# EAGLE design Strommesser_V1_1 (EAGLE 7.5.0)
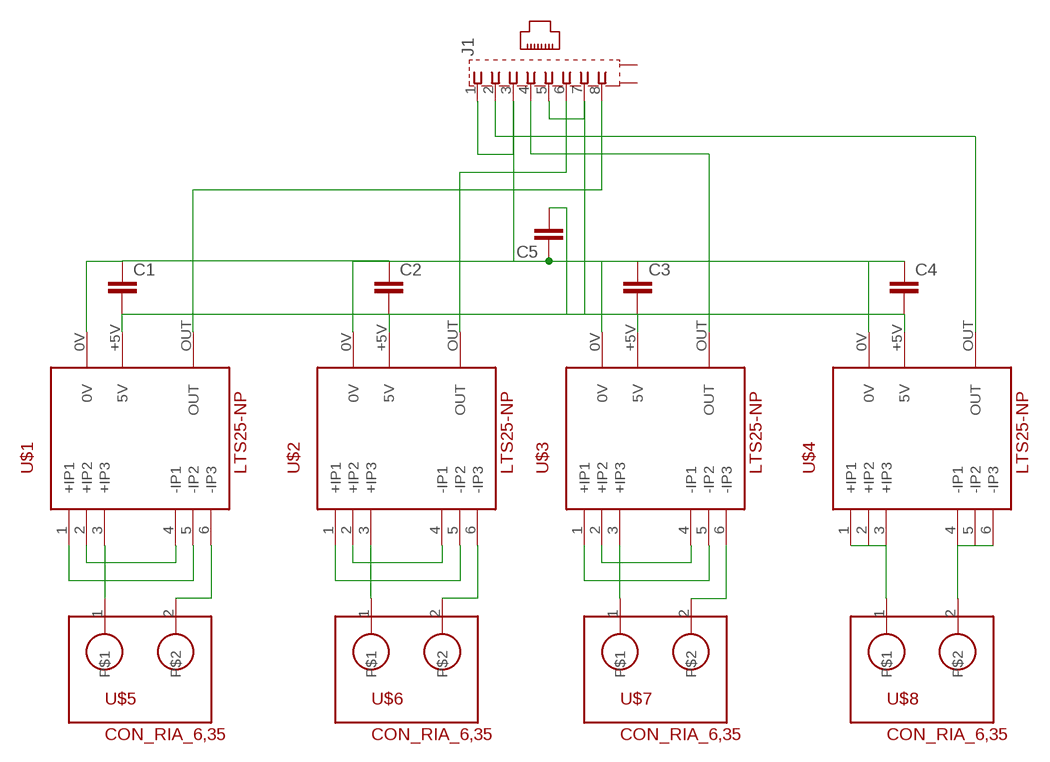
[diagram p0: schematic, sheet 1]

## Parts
C1  C-EUC0603  [C0603]
C2  C-EUC0603  [C0603]
C3  C-EUC0603  [C0603]
C4  C-EUC0603  [C0603]
C5  C-EUC1206  [C1206]
J1  557730-1  [557730-1]
U$1  LTS25-NP  [LTS]
U$2  LTS25-NP  [LTS]
U$3  LTS25-NP  [LTS]
U$4  LTS25-NP  [LTS]
U$5  CON_RIA_6,35  [CON_RIA6,35]
U$6  CON_RIA_6,35  [CON_RIA6,35]
U$7  CON_RIA_6,35  [CON_RIA6,35]
U$8  CON_RIA_6,35  [CON_RIA6,35]

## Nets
N$1: J1.8 U$1.OUT
N$2: J1.2 U$4.OUT
N$3: C1.1 C2.1 C3.1 C4.1 C5.1 J1.1 J1.3 U$1.0V U$2.0V U$3.0V U$4.0V
N$4: C1.2 C2.2 C3.2 C4.2 C5.2 J1.5 J1.7 U$1.+5V(5V) U$2.+5V(5V) U$3.+5V(5V) U$4.+5V(5V)
N$5: J1.4 U$3.OUT
N$6: J1.6 U$2.OUT
N$7: U$1.3(+IP3) U$5.1
N$8: U$1.2(+IP2) U$1.4(-IP1)
N$9: U$1.1(+IP1) U$1.5(-IP2)
N$10: U$1.6(-IP3) U$5.2
N$11: U$2.3(+IP3) U$6.1
N$12: U$3.3(+IP3) U$7.1
N$13: U$2.2(+IP2) U$2.4(-IP1)
N$14: U$2.1(+IP1) U$2.5(-IP2)
N$15: U$4.1(+IP1) U$4.2(+IP2) U$4.3(+IP3) U$8.1
N$16: U$4.4(-IP1) U$4.5(-IP2) U$4.6(-IP3) U$8.2
N$17: U$2.6(-IP3) U$6.2
N$18: U$3.2(+IP2) U$3.4(-IP1)
N$19: U$3.1(+IP1) U$3.5(-IP2)
N$20: U$3.6(-IP3) U$7.2
Unconnected: J1.G1(S2) J1.G2(S1)

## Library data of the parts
C1-C5 = rcl:C-EU: CAPACITOR, European symbol
J1 = con-amp:557730-1: AMP connector
U$1-U$4 = LTS25-NP:LTS25-NP
U$5-U$8 = con_Ria:CON_RIA_6,35

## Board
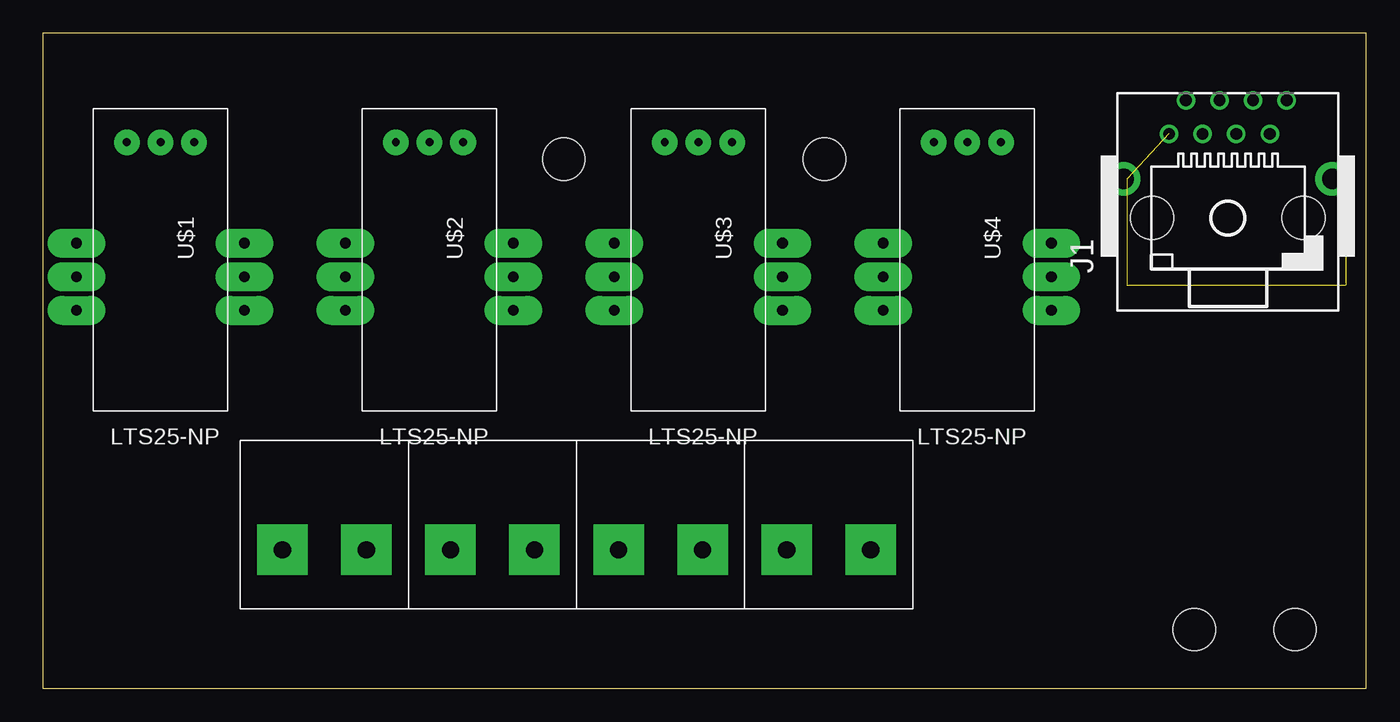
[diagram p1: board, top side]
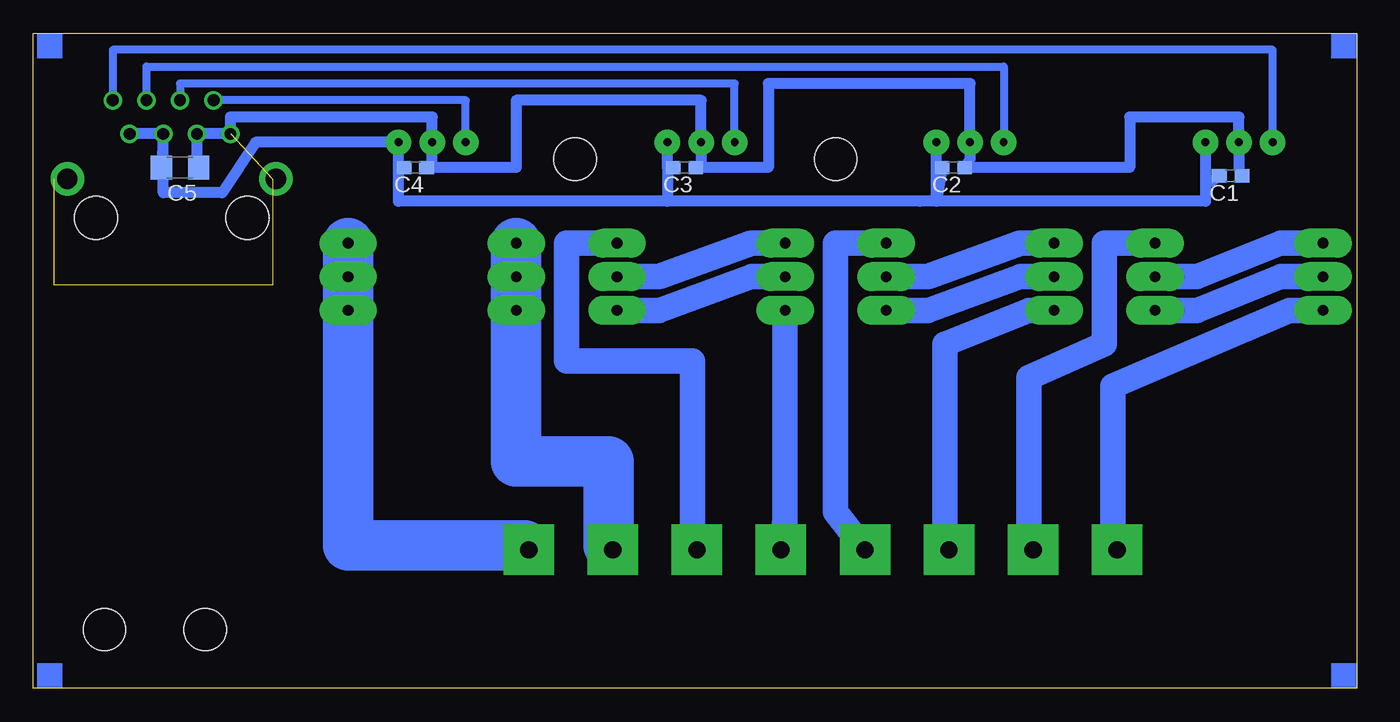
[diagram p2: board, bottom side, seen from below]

Size 100 x 49.52 mm. Coordinates in mm from the lower left corner, seen from the top.
Outline: 0,0 100,0 100,49.52 0,49.52 0,0
Copper layers (1*16): Top 0.035mm / dielectric 1.5mm / Bottom 0.035mm
Design rules "default": minimum track width 10mil, minimum drill 24mil, track to track 8mil, track to pad 8mil, pad to pad 8mil, via to via 8mil, smd to smd 8mil, copper to edge 40mil, drill to drill 8mil, minimum pad ring 10mil, minimum via ring 8mil, stop-mask expansion 4mil, vias tented up to drill 0mil, thermal gap 10mil
Holes 3.2 mm at 94.61,4.45 87,4.45 59.05,40.01 39.37,40.01

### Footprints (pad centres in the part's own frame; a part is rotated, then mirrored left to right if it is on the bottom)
C0603 = smd 1.1 x 1: 1 -0.85,0; 2 0.85,0
C1206 = smd 1.6 x 1.8: 1 -1.4,0; 2 1.4,0
557730-1 = drill 0.889: 1 -4.445,6.35; 2 -3.175,8.89; 3 -1.905,6.35; 4 -0.635,8.89; 5 0.635,6.35; 6 1.905,8.89; 7 3.175,6.35; 8 4.445,8.89 | drill 1.524 pad 2.54: G1 -7.874,2.946; G2 7.874,2.946 | hole 3.251: -5.715,0; 5.715,0
LTS = drill 0.6 pad 1.93: 0V -10.16,0; +5V -10.16,2.54; OUT -10.16,-2.54 | drill 0.8 pad 2.184 long: 1 -2.54,-6.35; 2 0,-6.35; 3 2.54,-6.35; 4 2.54,6.35; 5 0,6.35; 6 -2.54,6.35
CON_RIA6,35 = drill 1.3 pad 3.81 square: 1 -3.493,-1.587; 2 2.857,-1.587

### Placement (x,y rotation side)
C1  9.53,38.73 180 bottom
C2  30.48,39.37 180 bottom
C3  50.8,39.37 180 bottom
C4  71.12,39.37 180 bottom
C5  88.9,39.37 180 bottom
J1  89.53,35.56 0 top
U$1  8.89,31.11 270 top
U$2  29.21,31.11 270 top
U$3  49.53,31.11 270 top
U$4  69.85,31.11 270 top
U$5  21.59,12.06 0 top
U$6  34.29,12.06 0 top
U$7  46.99,12.06 0 top
U$8  59.69,12.06 0 top

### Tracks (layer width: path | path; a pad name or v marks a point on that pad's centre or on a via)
N$1
  Bottom 0.61: U$1.OUT 6.35,48.26 93.98,48.26 J1.8
N$2
  Bottom 0.61: U$4.OUT 67.31,44.45 J1.2
N$3  (4 unrouted)
  Bottom 0.813: C1.1 8.89,39.37 U$1.0V 8.89,43.18 17.14,43.18 17.14,39.37 C2.1 29.21,40.01 U$2.0V 29.21,45.72 44.45,45.72 44.45,39.37 49.53,39.37 | 49.53,39.37 C3.1 | 49.53,39.37 U$3.0V 49.53,44.45 63.5,44.45 63.5,39.37 69.85,39.37 | C5.1 87.63,40.01 J1.3 J1.1 85.09,43.18 69.85,43.18 U$4.0V 69.85,39.37 | 69.85,39.37 C4.1
N$4
  Bottom 0.813: U$1.+5V 11.43,38.1 | 11.43,38.1 C1.2 | 11.43,38.1 11.43,36.83 31.75,36.83 | 31.75,36.83 U$2.+5V | C2.2 31.75,36.83 | 31.75,36.83 33.02,36.83 52.07,36.83 | 52.07,39.37 U$3.+5V | C3.2 52.07,39.37 | 52.07,39.37 52.07,36.83 | 52.07,36.83 72.39,36.83 72.39,39.37 | C4.2 72.39,39.37 | 72.39,39.37 U$4.+5V 83.19,41.27 85.72,37.47 90.17,37.47 J1.5 | J1.5 J1.7 | J1.5 C5.2
N$5
  Bottom 0.61: U$3.OUT 46.99,45.72 88.9,45.72 J1.4
N$6
  Bottom 0.61: U$2.OUT 26.67,46.99 91.44,46.99 J1.6
N$7
  Bottom 1.93: U$1.3 5.08,28.57 18.41,22.86 18.41,10.79 U$5.1
N$8
  Bottom 1.93: U$1.2 5.71,31.11 12.06,28.57 U$1.4
N$9
  Bottom 1.93: U$1.1 5.71,33.66 12.06,31.11 U$1.5
N$10
  Bottom 1.93: U$1.6 19.05,33.66 19.05,26.04 24.77,23.5 24.77,12.06 U$5.2
N$11
  Bottom 1.93: U$2.3 24.77,28.57 31.11,26.04 31.11,10.79 U$6.1
N$12
  Bottom 1.93: U$3.3 43.18,12.7 U$7.1
N$13
  Bottom 1.93: U$2.2 25.4,31.11 32.38,28.57 U$2.4
N$14
  Bottom 1.93: U$2.1 25.4,33.66 32.38,31.11 U$2.5
N$15
  Bottom 2.54: U$4.1 U$4.2 U$4.3
  Bottom 3.81: U$4.1 U$4.3 63.5,17.14 56.52,17.14 56.52,10.79 U$8.1
N$16
  Bottom 2.54: U$4.6 U$4.5 U$4.4
  Bottom 3.81: U$4.4 U$4.6 76.2,10.79 62.87,10.79 U$8.2
N$17
  Bottom 1.93: U$2.6 39.37,33.66 39.37,13.34 U$6.2
N$18
  Bottom 1.93: U$3.2 45.72,31.11 52.7,28.57 U$3.4
N$19
  Bottom 1.93: U$3.1 45.72,33.66 52.7,31.11 U$3.5
N$20
  Bottom 1.93: U$3.6 59.69,33.66 59.69,24.77 50.16,24.77 50.16,10.79 U$7.2
(copper drawn outside any net)
  shapes: Bottom area x4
